// ----------------------------------------------------------------------------
// S7 DEMO PROGRAM FOR ONE FTP CLIENT CONNECTION
//
// This program performs the following actions in an endless loop as long as
// no error occurs:
//      FTP_CONNECT  (FC40)
//      FTP_RETRIEVE (FC42)
//      FTP_QUIT     (FC44)
//
// The code is located in FC1. It is called in OB35.
// To use this simple demo successfully, follow the steps below:
//
// 1.) Use STEP 7 V5.1 ServicePack 3 (or higher) and create a project with
//     at least 1 CPU and 1 IT-CP (6GK7 343/443-1GX11-0XE0 or higher)
//
// 2.) Create a FTP client connection by opening NetPro and creating an
//     unspecified TCP connection and checking the option 'Use FTP protocol'.
//     Enter the ID of this connection at the beginning of FC1. See also
//     comment: "user modification (1)"
//
// 3.) Obtain the LADDR of your IT-CP and enter this value at the beginning of
//     FC1. See comment: "user modification (2)"
//
// 4.) Some modification is required in DB40. This DB defines the login
//     properties for the FTP server and the file that will be retrieved
//     in this example.
//
// 5.) Run an FTP server on a network that can be reached by your IT-CP.
//     Create a small file (a few hundred bytes) with the name you specified
//     in DB40. Place it in the root of the user you also specified in DB40.
//
// 6.) Copy UDT1 and the FCs FC40 - FC44 from the SIMATIC_NET_CP library and
//     insert them in your project. If you use a CP343-1 IT you will also
//     have to copy the FC 5 from the library. Compile this source, download
//     FC40 - FC44 (and eventually FC 5) and all the objects created from
//     this source to the CPU. These objects are: DB9, DB40, DB42, FC1, OB35.
//     The compiler should not report any errors or warnings.
//     Set MW200 to 0 to start the sequence.
//
// ----------------------------------------------------------------------------

DATA_BLOCK DB40
NAME : FTP_DATA
STRUCT
   ip_addr   : STRING [100];    // Do not change the lengths
   user      : STRING [32];     // of the following items.
   password  : STRING [32];     //
   file_name : STRING [220];    //
END_STRUCT;
BEGIN
   ip_addr   := '142.11.41.50'; // IP address, user and password of the
   user      := 'eric';         // FTP server that will be used in this
   password  := 'clapton';      // example. Modify the items to match
   file_name := 'testfile.dat'; // your environment.
END_DATA_BLOCK

// ----------------------------------------------------------------------------

DATA_BLOCK DB42
NAME : FTP_FILE
STRUCT
   hdr            : UDT 1;
   filedata       : ARRAY [0 .. 999] OF BYTE;
END_STRUCT;
BEGIN
   hdr.exist      := FALSE;   // is set after the first FTP_RETRIEVE
   hdr.locked     := FALSE;   // temp. is set and reset by FTP_RETRIEVE
   hdr.new        := FALSE;   // is set after every FTP_RETRIEVE. Manual reset is necessary.
   hdr.writeaccess:= FALSE;   // write access: FALSE-->for FTP client on IT-CP, TRUE-->for server on IT-CP
   hdr.act_length := L#0;     // is set by FTP_RETRIEVE
   hdr.max_length := L#1000;  // initial value; change only if size of array "filedata" is changed.
END_DATA_BLOCK

// ----------------------------------------------------------------------------

DATA_BLOCK DB9
NAME : FTP_BUFFER
STRUCT
   reserved : ARRAY [0 .. 255] OF BYTE;
END_STRUCT;
BEGIN
END_DATA_BLOCK

// ----------------------------------------------------------------------------

FUNCTION FC1: VOID
NAME : FTPCdemo
BEGIN
NETWORK
//To start, set MW200 to 0 in a VAT
    SET;
// ------------------------------------------- user modification (1) ----------
    L 1;            // Load connection ID of the FTP connection and store it
    T MW 202;       // in MW202 for use in the FTP function calls
// ------------------------------------------- user modification (2) ----------
    L 520;          // Load LADDR of your IT-CP and store it
    T MW 204;       // in MW204 for use in the FTP function calls
// ----------------------------------------------------------------------------
    S M 210.0;      // ACT:=1 for FTP_CONNECT, FTP_RETRIEVE and FTP_QUIT.
    S M 220.0;      // Never call the FTP_xxx funtions with ACT:=0,
    S M 230.0;      // this will cause an error with STATUS 0x8F70 !
// ----------------------------------------------------------------------------
    L MW 200;       // This is a simple state machine so that commands
    L 0;            // are executed in the right order.
    ==I;            //
    JC conn;        // Initiate or poll FTP_CONNECT
// ----------------------------------------------------------------------------
    L MW 200;       //
    L 1;            //
    ==I;            //
    JC retr;        // Initiate or poll FTP_RETRIEVE
// ----------------------------------------------------------------------------
    L MW 200;       //
    L 2;            //
    ==I;            //
    JC quit;        // Initiate or poll FTP_QUIT
// ----------------------------------------------------------------------------
    JU end;         // Not a legal value for MW200, so do nothing.
                    // By setting MW200 to 0, the command sequence will start again
                    // and connect to the specified FTP server
// ----------------------------------------------------------------------------
conn: CALL "FTP_CONNECT" (
        ACT          := M 210.0,
        ID           := MW 202,
        LADDR        := MW 204,
        LOGIN        := P#DB40.DBX 0.0 BYTE 170,
        BUFFER_DB_NR := 9,
        DONE         := M 210.1,
        ERROR        := M 210.2,
        STATUS       := MW 212
      );
// ----------------------- if ( error == 1 ) ----------------------------------
    SET;            // { Run a simple error routine. (An extended error routine
    A M 210.2;      //   could repeat the connect command if the error code is
    JC err;         //   0x8F61 : FTP server is off;  0x8F6A : temporary no resource on IT-CP) }
// ----------------------- if ( done == 0 ) -----------------------------------
    SET;            // {
    AN M 210.1;     //   Poll again next cycle
    JC end;         // }
// ----------------------- else -----------------------------------------------
    L 1;            // { Set MW200 so that the program activates the RETRIEVE command
    T MW 200;       //   in the next cycle. This allows an FTP_RETRIEVE command on this DB.
    R DB42.hdr.new; // }
// ----------------------------------------------------------------------------
retr: CALL "FTP_RETRIEVE" (
        ACT          := M 220.0,
        ID           := MW 202,
        LADDR        := MW 204,
        FILE_NAME    := P#DB40.DBX 170.0 BYTE 222,
        BUFFER_DB_NR := 9,
        FILE_DB_NR   := 42,
        DONE         := M 220.1,
        ERROR        := M 220.2,
        STATUS       := MW 222
      );
// ----------------------- if ( error == 1 ) ----------------------------------
    SET;            // {
    A M 220.2;      //   Run a simple error routine
    JC err;         // }
// ----------------------- if ( done == 0 ) -----------------------------------
    SET;            // {
    AN M 220.1;     //   Poll again next cycle
    JC end;         // }
// ----------------------- else -----------------------------------------------
    L 2;            // { Set MW200 so that the program activates
    T MW 200;       //   the FTP_QUIT command in the next cycle }
// ----------------------------------------------------------------------------
quit: CALL "FTP_QUIT" (
        ACT    := M 230.0,
        ID     := MW 202,
        LADDR  := MW 204,
        DONE   := M 230.1,
        ERROR  := M 230.2,
        STATUS := MW 232
      );
// ----------------------- if ( error == 1 ) ----------------------------------
    SET;            // {
    A M 230.2;      //   Run a simple error routine
    JC err;         // }
// ----------------------- if ( done == 0 ) -----------------------------------
    SET;            // {
    AN M 230.1;     //   Poll again next cycle
    JC end;         // }
// ----------------------- else -----------------------------------------------
    L 0;            // { Set MW200 so that the program activates
    T MW 200;       //   the FTP_CONNECT command in the next cycle
    JU end;         // }
// ----------------------------------------------------------------------------
err: L 255;         // This is the error exit for FC1. MW200 is set to 255.
    T MW 200;       // After this, the state machine will not execute any more
                    // FTP_xxx calls. Setting MW200 to 0 starts the sequence again.
// ----------------------------------------------------------------------------
end: BEU;
END_FUNCTION

// ----------------------------------------------------------------------------

ORGANIZATION_BLOCK OB 35
TITLE = FTP_TRIGGER
VAR_TEMP
   OB35_EV_CLASS : BYTE;           // Bits 0-3 = 1 (Coming event), Bits 4-7 = 1 (Event class 1)
   OB35_STRT_INF : BYTE;           // 16#36 (OB 35 has started)
   OB35_PRIORITY : BYTE;           // Priority of OB Execution
   OB35_OB_NUMBR : BYTE;           // 35 (Organization block 35, OB35)
   OB35_RESERVED_1 : BYTE;         // Reserved for system
   OB35_RESERVED_2 : BYTE;         // Reserved for system
   OB35_PHASE_OFFSET : WORD;       // Phase offset (msec)
   OB35_RESERVED_3 : INT;          // Reserved for system
   OB35_EXC_FREQ : INT;            // Frequency of execution (msec)
   OB35_DATE_TIME : DATE_AND_TIME; // Date and time OB35 started
END_VAR
BEGIN
NETWORK
   call FC1;
END_ORGANIZATION_BLOCK

// ----------------------------------------------------------------------------
